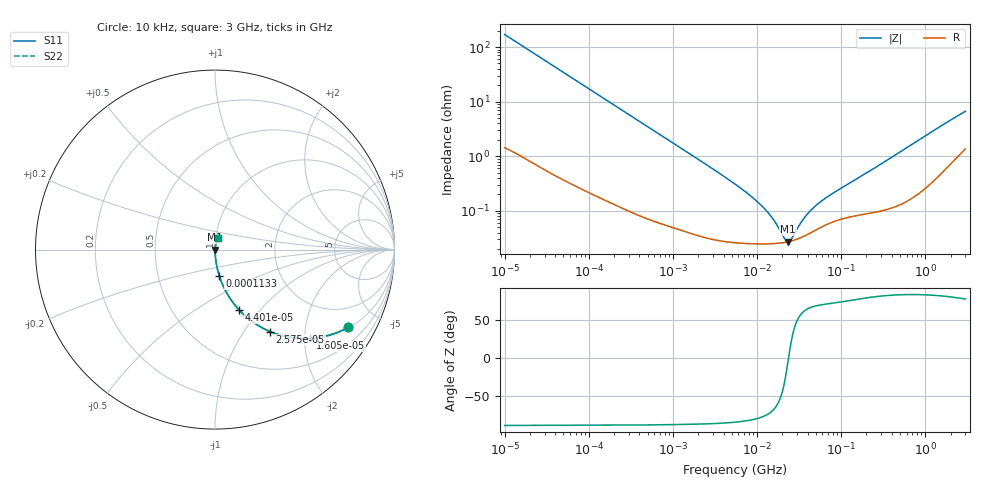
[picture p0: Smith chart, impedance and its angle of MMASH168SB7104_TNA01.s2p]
! MMASH168SB7104_TNA01  S-PARAMETER MODEL  ( Standard Model )
! Model Generated by TAIYO YUDEN Corporation (http://www.ty-top.com)
! Version 1.0
! TAIYO YUDEN Control No. 220601
! Copyright(c) 2015 TAIYO YUDEN CO.,LTD. All Rights Reserved.
! Product Description (link to TY-COMPAS)
! https://ds.yuden.co.jp/TYCOMPAS/or/detail?pn=MMASH168SB7104KTNA01&u=M
! Products Name : Multilayer Ceramic Capacitors
! Characteristics :
!  Capacitance : 0.1 [uF] , Rated Voltage : 100 [V] , TCC : X7R
!  Case Size : 1.6 x 0.8 / 0.063 x 0.031 [mm/inch] , Thickness : 0.8 / 0.031 [mm/inch]
!  (Conditions: Temperature = 25 [degC] , DC Bias Voltage = 0 [V])
! External Node Assignments :
!  1  o---| |---o  2
! GND o---------o GND
! Frequency Range : 10kHz  -  3GHz  [ 401 STEP ]
# MHZ S RI R 50
! Freq[MHz].  S11 Real  S11 Imag  S21 Real  S21 Imag  S12 Real  S12 Imag  S22 Real  S22 Imag
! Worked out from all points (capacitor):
!   401 points, 10 kHz to 3 GHz, reference 50 ohm
!   read as one part in series: C = 93.5 nF near 10.65 kHz
!   lowest |Z| = 27.3 mohm at 23.36 MHz (marker M1)
!   series resonance near 23.71 MHz, so ESL is about 480 pH
!   S11 on the Smith chart (normalised r, x): 10 kHz: 1.03, -3.40; 16.05 kHz: 1.02, -2.12; 25.75 kHz: 1.01, -1.33; 44.01 kHz: 1.01, -0.78; 113.3 kHz: 1.00, -0.30; 3 GHz: 1.03, +0.13
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0.01  0.7409 -0.434  0.2591 0.434  0.2591 0.434  0.7409 -0.434
0.016047  0.5297 -0.4945  0.4703 0.4945  0.4703 0.4945  0.5297 -0.4945
0.02575  0.3075 -0.4567  0.6925 0.4567  0.6925 0.4567  0.3075 -0.4567
0.044011  0.1343 -0.3358  0.8657 0.3358  0.8657 0.3358  0.1343 -0.3358
0.082683  0.0437 -0.1985  0.9563 0.1985  0.9563 0.1985  0.0437 -0.1985
0.11333  0.0245 -0.1482  0.9755 0.1482  0.9755 0.1482  0.0245 -0.1482
0.249268  0.00593 -0.0691  0.9941 0.0691  0.9941 0.0691  0.00593 -0.0691
0.683653  0.00125 -0.0255  0.9987 0.0255  0.9987 0.0255  0.00125 -0.0255
5.477226  0.00027 -0.00308  0.9997 0.00308  0.9997 0.00308  0.00027 -0.00308
8.789267  0.000253 -0.00176  0.9997 0.00176  0.9997 0.00176  0.000253 -0.00176
12.43293  0.000249 -0.00105  0.9998 0.00105  0.9998 0.00105  0.000249 -0.00105
15.99985  0.000252 -0.000612  0.9997 0.000612  0.9997 0.000612  0.000252 -0.000612
21.24962  0.000264 -0.000167  0.9997 0.000167  0.9997 0.000167  0.000264 -0.000167
23.35767  0.000272 -2.27e-05  0.9997 2.27e-05  0.9997 2.27e-05  0.000272 -2.27e-05
25.67485  0.000282 0.00012  0.9997 -0.00012  0.9997 -0.00012  0.000282 0.00012
34.09912  0.00033 0.000554  0.9997 -0.000554  0.9997 -0.000554  0.00033 0.000554
45.28751  0.000412 0.001  0.9996 -0.001  0.9996 -0.001  0.000412 0.001
56.47134  0.000494 0.00137  0.9995 -0.00137  0.9995 -0.00137  0.000494 0.00137
75.00035  0.000606 0.00188  0.9994 -0.00188  0.9994 -0.00188  0.000606 0.00188
374.4521  0.00117 0.00892  0.9988 -0.00892  0.9988 -0.00892  0.00117 0.00892
1596.854  0.00637 0.0365  0.9936 -0.0365  0.9936 -0.0365  0.00637 0.0365
3000  0.0175 0.0631  0.9825 -0.0631  0.9825 -0.0631  0.0175 0.0631
